(* Logix 5000 DataType export EdDSA_STATECTRL; software revision 30.00 *)

TYPE EdDSA_STATECTRL :
STRUCT
   RESET : BOOL;
   DN : BOOL;
   START : BOOL;
   ONS : INT;
   STEP : INT;
   CMD : INT;
   CMD_TABLE : INT[20];
   DONE : INT;
   NEXT_STEP : INT;
   TIMER : TIMER[5];
   NEXT_STATE : INT;
   TEMP : DINT[5];
END_STRUCT
END_TYPE
